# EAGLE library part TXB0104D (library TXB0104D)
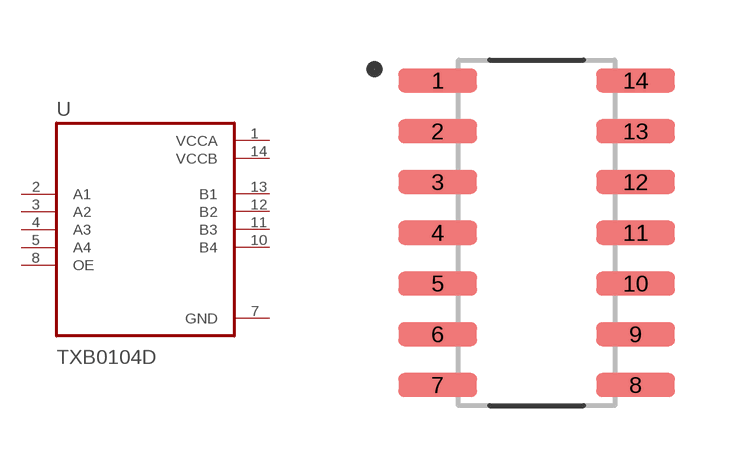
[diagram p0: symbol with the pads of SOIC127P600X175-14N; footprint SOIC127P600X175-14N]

Designator prefix U

## TXB0104D (Check_prices: https://www.snapeda.com/parts/TXB0104D/Texas+Instruments/view-part/?ref=eda; Description: 4-Bit Bidirectional Voltage-Level Shifter with Auto Direction Sensing and +/-15 kV ESD Protect; MF: Texas Instruments; MP: TXB0104D; Package: SOIC-14 Texas Instruments; Purchase-URL: https://www.snapeda.com/api/url_track_click_mouser/?unipart_id=44550&manufacturer=Texas Instruments&part_name=TXB0104D&search_term=txb0104; RS_Components_7092778P_Purchase_URL: https://www.snapeda.com/api/url_track_click/https%253A//uk.rs-online.com/web/p/translator-ics/7092778p//%253Futm_campaign%253Dbuynow%2526utm_medium%253Daggregator%2526utm_source%253Dsnapeda%2526cm_mmc%253Daff-_-uk-_-snapeda-_-7092778P/?unipart_id=44550&manufacturer=Texas Instruments&part_name=TXB0104D&search_term=txb0104; RS_Components_7092778_Purchase_URL: https://www.snapeda.com/api/url_track_click/https%253A//uk.rs-online.com/web/p/translator-ics/7092778//%253Futm_campaign%253Dbuynow%2526utm_medium%253Daggregator%2526utm_source%253Dsnapeda%2526cm_mmc%253Daff-_-uk-_-snapeda-_-7092778/?unipart_id=44550&manufacturer=Texas Instruments&part_name=TXB0104D&search_term=txb0104; RS_Components_9236790_Purchase_URL: https://www.snapeda.com/api/url_track_click/https%253A//uk.rs-online.com/web/p/translator-ics/9236790//%253Futm_campaign%253Dbuynow%2526utm_medium%253Daggregator%2526utm_source%253Dsnapeda%2526cm_mmc%253Daff-_-uk-_-snapeda-_-9236790/?unipart_id=44550&manufacturer=Texas Instruments&part_name=TXB0104D&search_term=txb0104; SnapEDA_Link: https://www.snapeda.com/parts/TXB0104D/Texas+Instruments/view-part/?ref=snap)  [SOIC127P600X175-14N]
1  VCCA  pwr
2  A1  in
3  A2  in
4  A3  in
5  A4  in
7  GND  pwr
8  OE  in
10  B4  out
11  B3  out
12  B2  out
13  B1  out
14  VCCB  pwr

## Footprint SOIC127P600X175-14N (pad centres in mm)
smd 1.97 x 0.6: 1 -2.475,3.81; 2 -2.475,2.54; 3 -2.475,1.27; 4 -2.475,0; 5 -2.475,-1.27; 6 -2.475,-2.54; 7 -2.475,-3.81; 8 2.475,-3.81; 9 2.475,-2.54; 10 2.475,-1.27; 11 2.475,0; 12 2.475,1.27; 13 2.475,2.54; 14 2.475,3.81

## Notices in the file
This work is licensed under a Creative Commons Attribution-ShareAlike 4.0 International License (CC BY-SA) with Design Exception 1.0
